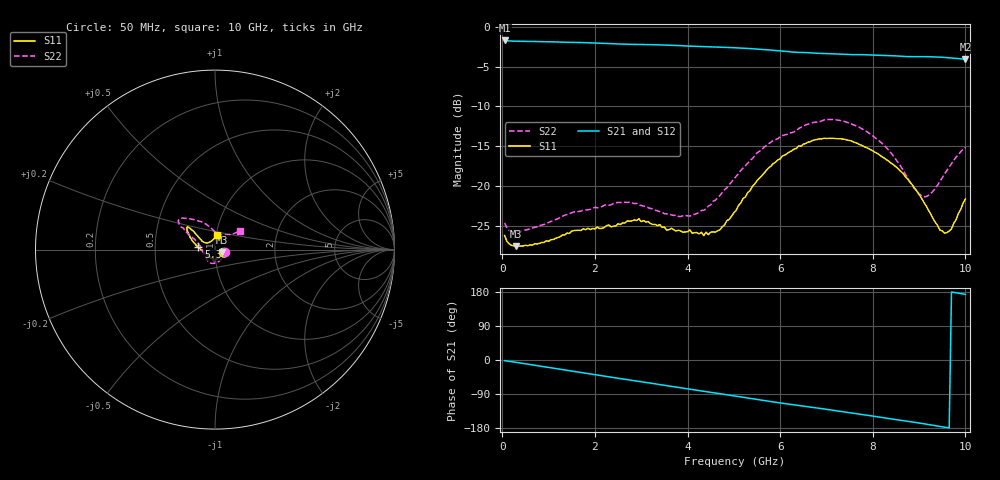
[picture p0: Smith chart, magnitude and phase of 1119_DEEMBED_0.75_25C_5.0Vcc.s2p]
!Hittite Microwave Corp.
!Digital Attenuator/PhaseShifter Rev 1.4.0
!Filename: C:\DATA\DATA\1119_DEEMBED_0.75_25C_5.0Vcc.s2p
!VNA ID: Agilent Technologies,N5224A,MY51441122,A.10.45.03
!Device type:
!2 Port Calibration.
!Temp(C): 25
!Lot Number:
!Serial Number:
!Operator:
!Misc:
!Attenuator:  0.750
# GHZ S DB R 50.0
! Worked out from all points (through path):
!   200 points, 50 MHz to 10 GHz, reference 50 ohm
!   highest |S21| = -1.72 dB at 50 MHz (marker M1); lowest = -4.1 dB at 10 GHz (marker M2)
!   group delay of S21, straight-line fit = 51 ps
!   lowest |S11| = -27.6 dB at 300 MHz (marker M3), VSWR 1.09, Z = 54.1 - j1.39 ohm
!   |S11| at or under -10 dB: start of sweep to end of sweep
!   |S22| runs from -25.7 to -11.6 dB; largest |S21 - S12| = 0.002
!   S11 on the Smith chart (normalised r, x): 50 MHz: 1.10, -0.03; 5.35 GHz: 0.83, +0.02; 10 GHz: 1.01, +0.17
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0.05  -26.22 -15.3  -1.72 -1.8  -1.72 -1.7  -24.63 -12.4
0.15  -27.28 -14.3  -1.78 -3.4  -1.78 -3.4  -25.58 -13.1
0.3  -27.56 -17.9  -1.81 -6.2  -1.81 -6.2  -25.74 -17.7
1.75  -25.37 -78.0  -1.99 -34.0  -1.98 -34.0  -23.05 -75.7
2.65  -24.64 -90.1  -2.19 -50.9  -2.19 -51.0  -22.03 -107.6
2.95  -24.12 -94.9  -2.21 -56.3  -2.22 -56.4  -22.40 -118.9
3.4  -24.86 -101.8  -2.27 -64.8  -2.27 -64.8  -23.20 -133.8
3.85  -25.64 -108.3  -2.38 -73.3  -2.38 -73.3  -23.84 -149.7
4.35  -26.24 -125.8  -2.49 -82.5  -2.50 -82.5  -23.05 -177.5
4.7  -25.50 -149.9  -2.57 -89.0  -2.59 -89.1  -21.19 165.7
5.05  -23.06 -174.0  -2.65 -95.5  -2.66 -95.6  -18.79 155.4
5.35  -20.59 171.3  -2.74 -101.3  -2.75 -101.4  -16.81 151.7
6.05  -16.22 154.2  -3.06 -114.2  -3.08 -114.3  -13.67 146.5
6.7  -14.29 144.4  -3.29 -125.1  -3.30 -125.1  -12.05 143.7
7.45  -14.24 140.4  -3.47 -138.1  -3.48 -138.1  -12.01 135.6
7.9  -15.27 139.5  -3.53 -146.1  -3.54 -146.2  -13.29 128.1
8.35  -16.91 140.4  -3.62 -154.4  -3.62 -154.4  -15.55 114.4
8.9  -20.25 145.7  -3.75 -164.3  -3.75 -164.3  -20.33 89.3
9.15  -22.48 146.9  -3.76 -169.2  -3.77 -169.2  -21.34 72.2
9.55  -25.93 123.2  -3.86 -177.4  -3.87 -177.4  -18.48 45.1
9.7  -25.37 105.1  -3.92 179.5  -3.93 179.5  -17.20 40.3
10  -21.64 81.4  -4.08 173.2  -4.08 173.2  -15.16 37.1
